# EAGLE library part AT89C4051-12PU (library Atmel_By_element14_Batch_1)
Microcontroller
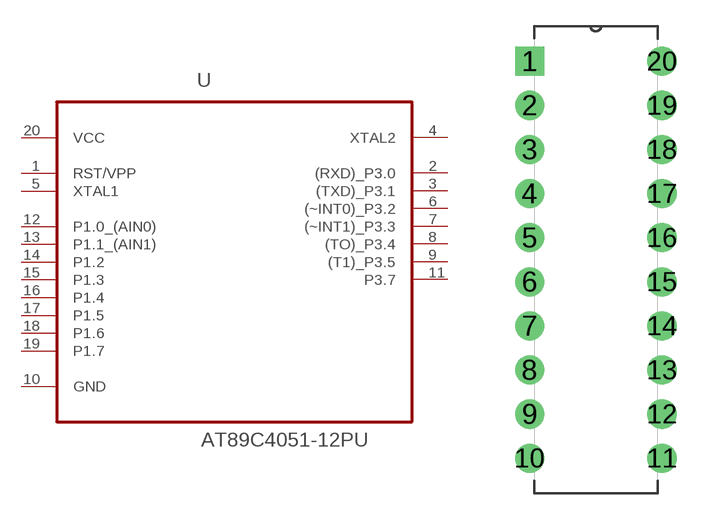
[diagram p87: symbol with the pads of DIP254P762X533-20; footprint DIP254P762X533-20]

Designator prefix U

## AT89C4051-12PU (DESCRIPTION: Microcontroller; MPN: AT89C4051-12PU; OC_FARNELL: 1699391; OC_NEWARK: 80P3689; PACKAGE: DIP-20; SUPPLIER: ATMEL)  [DIP254P762X533-20]
1  RST/VPP  pwr
2  (RXD)_P3.0
3  (TXD)_P3.1
4  XTAL2  out
5  XTAL1  in
6  (~INT0)_P3.2
7  (~INT1)_P3.3
8  (TO)_P3.4
9  (T1)_P3.5
10  GND  pas
11  P3.7
12  P1.0_(AIN0)
13  P1.1_(AIN1)
14  P1.2
15  P1.3
16  P1.4
17  P1.5
18  P1.6
19  P1.7
20  VCC  pwr

## Footprint DIP254P762X533-20 (pad centres in mm)
drill 1.118 square: 1 -7.62,22.86
drill 1.118: 2 -7.62,20.32; 3 -7.62,17.78; 4 -7.62,15.24; 5 -7.62,12.7; 6 -7.62,10.16; 7 -7.62,7.62; 8 -7.62,5.08; 9 -7.62,2.54; 10 -7.62,0; 11 0,0; 12 0,2.54; 13 0,5.08; 14 0,7.62; 15 0,10.16; 16 0,12.7; 17 0,15.24; 18 0,17.78; 19 0,20.32; 20 0,22.86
